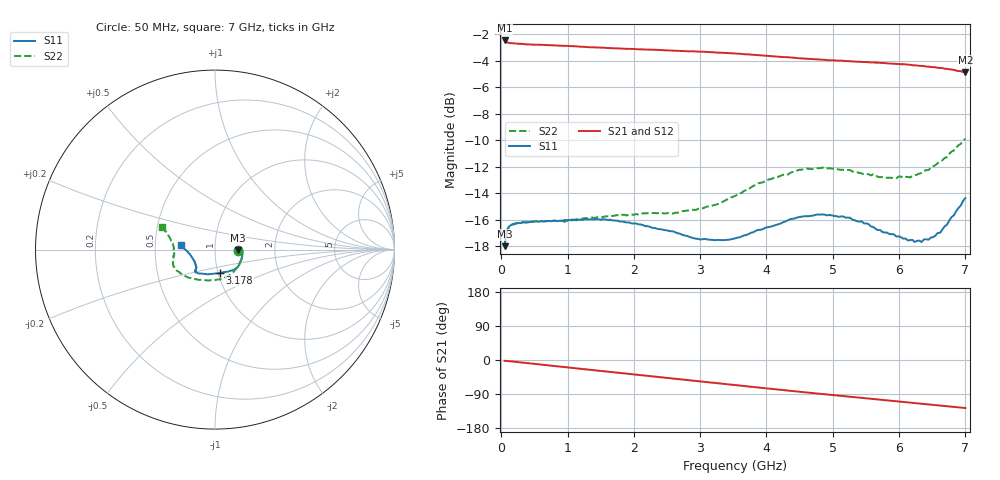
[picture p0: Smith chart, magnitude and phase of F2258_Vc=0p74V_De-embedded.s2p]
! Integrated Device Technology
! Corporate Headquarters
! 6024 Silver Creek Valley Road
! San Jose, CA 95138  USA
! Phone:  1-408-284-8200
! Toll Free:  1-800-223-1366
! Webpage:  http://www.idt.com/
! Timing and RF Division
! 515 Groton Road, Suite 102
! Westford, MA 01886-6024
! Device:  F2258
! Description: Voltage Variable RF Attenuator
! Frequency:  50.0 -  6000.00 MHz
! Package:  3x3 mm Thin QFN Plastic Package: 16 pin
! Ports:  2 RF, 2 DC
!  Pin  1  = NC
!  Pin  2  = NC
!  Pin  3  = RF2  = Port 2
!  Pin  4  = GND
!  Pin  5  = Vdd
!  Pin  6  = NC
!  Pin  7  = VCTRL
!  Pin  8  = NC
!  Pin  9  = GND
!  Pin 10  = RF1  = Port 1
!  Pin 11  = NC
!  Pin 12  = NC
!  Pin 13  = NC
!  Pin 14  = NC
!  Pin 15  = NC
!  Pin 16  = NC
! Vcntrl:  0.740 Volts
! Vdd:  +3.300 Volts
! Current:  1.125 mA
! Data:  The device was measured on a the F2258 evaluation board which has
!  individual transmission lines to the RF pins.  Data was collected
!  using a calibrated network analyzer.  The evaluation board was
!  de-embedded using a TRL calibration technique.
!  The reference plane is the edge of the package pin.
! Misc:  SN 10
!  Action Tracker AT0285
! Date Measured:  2014-12-10
! Date:  2016-01-13  MJV
! Note:
!  Integrated Device Technology supplies this data as a sample of measured
!  data at the package pin for this product.  Your particular data for this
!  product may vary.
!  Data was taken at 25 degrees C.
!  Integrated Device Technology reserves the right to change this data at anytime.
!Freq_(GHz)  S11M_(dB)  S11P_(deg)  S21M_(dB)  S21P_(deg)  S12M_(dB)  S12P_(deg)  S22M_(dB)  S22P_(deg)
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# GHz S dB R 50
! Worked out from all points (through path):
!   201 points, 50 MHz to 7 GHz, reference 50 ohm
!   highest |S21| = -2.48 dB at 50 MHz (marker M1); lowest = -4.9 dB at 7 GHz (marker M2)
!   group delay of S21, straight-line fit = 50.2 ps
!   lowest |S11| = -18.0 dB at 50 MHz (marker M3), VSWR 1.29, Z = 64.4 - j0.583 ohm
!   |S11| at or under -10 dB: start of sweep to end of sweep
!   |S22| runs from -17.8 to -9.9 dB; largest |S21 - S12| = 0.0031
!   S11 on the Smith chart (normalised r, x): 50 MHz: 1.29, -0.01; 3.178 GHz: 1.02, -0.27; 7 GHz: 0.68, +0.03
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0.05  -17.98 -2.0  -2.48 -2.1  -2.50 -2.1  -17.82 -2.5
0.08475  -16.85 -2.9  -2.61 -2.5  -2.63 -2.6  -16.75 -3.6
0.15425  -16.37 -4.4  -2.69 -3.7  -2.70 -3.7  -16.36 -6.5
0.50175  -16.13 -13.8  -2.80 -10.2  -2.83 -10.2  -16.08 -19.3
0.9535  -16.02 -27.2  -2.89 -18.8  -2.88 -18.8  -16.15 -37.5
1.2315  -16.00 -33.3  -2.96 -23.9  -2.97 -23.9  -15.90 -47.0
1.6485  -15.99 -41.1  -3.05 -31.5  -3.06 -31.5  -15.71 -59.6
2.37825  -16.70 -53.4  -3.20 -44.6  -3.20 -44.6  -15.49 -79.6
2.58675  -16.86 -58.0  -3.25 -48.5  -3.23 -48.5  -15.53 -86.1
2.93425  -17.42 -68.6  -3.30 -54.9  -3.31 -54.9  -15.25 -98.4
3.1775  -17.50 -77.7  -3.36 -59.5  -3.36 -59.5  -14.93 -107.9
3.525  -17.39 -93.4  -3.46 -66.0  -3.45 -66.0  -14.20 -122.0
4.0115  -16.56 -113.6  -3.64 -75.1  -3.63 -75.1  -12.99 -139.1
4.498  -15.79 -126.4  -3.83 -83.8  -3.82 -83.8  -12.22 -151.9
4.7065  -15.68 -128.7  -3.89 -87.5  -3.88 -87.4  -12.16 -156.1
5.2625  -15.85 -133.5  -4.06 -97.0  -4.06 -97.0  -12.25 -165.3
5.85325  -17.08 -138.7  -4.22 -107.1  -4.22 -107.1  -12.83 -176.5
6.166  -17.53 -146.3  -4.32 -112.6  -4.32 -112.6  -12.81 176.5
6.2355  -17.67 -149.8  -4.35 -113.8  -4.35 -113.8  -12.64 174.5
6.444  -17.50 -159.5  -4.46 -117.4  -4.44 -117.5  -12.25 169.4
6.61775  -16.97 -170.1  -4.56 -120.5  -4.55 -120.5  -11.64 164.7
7  -14.37 172.7  -4.89 -126.8  -4.86 -126.8  -9.88 156.5
